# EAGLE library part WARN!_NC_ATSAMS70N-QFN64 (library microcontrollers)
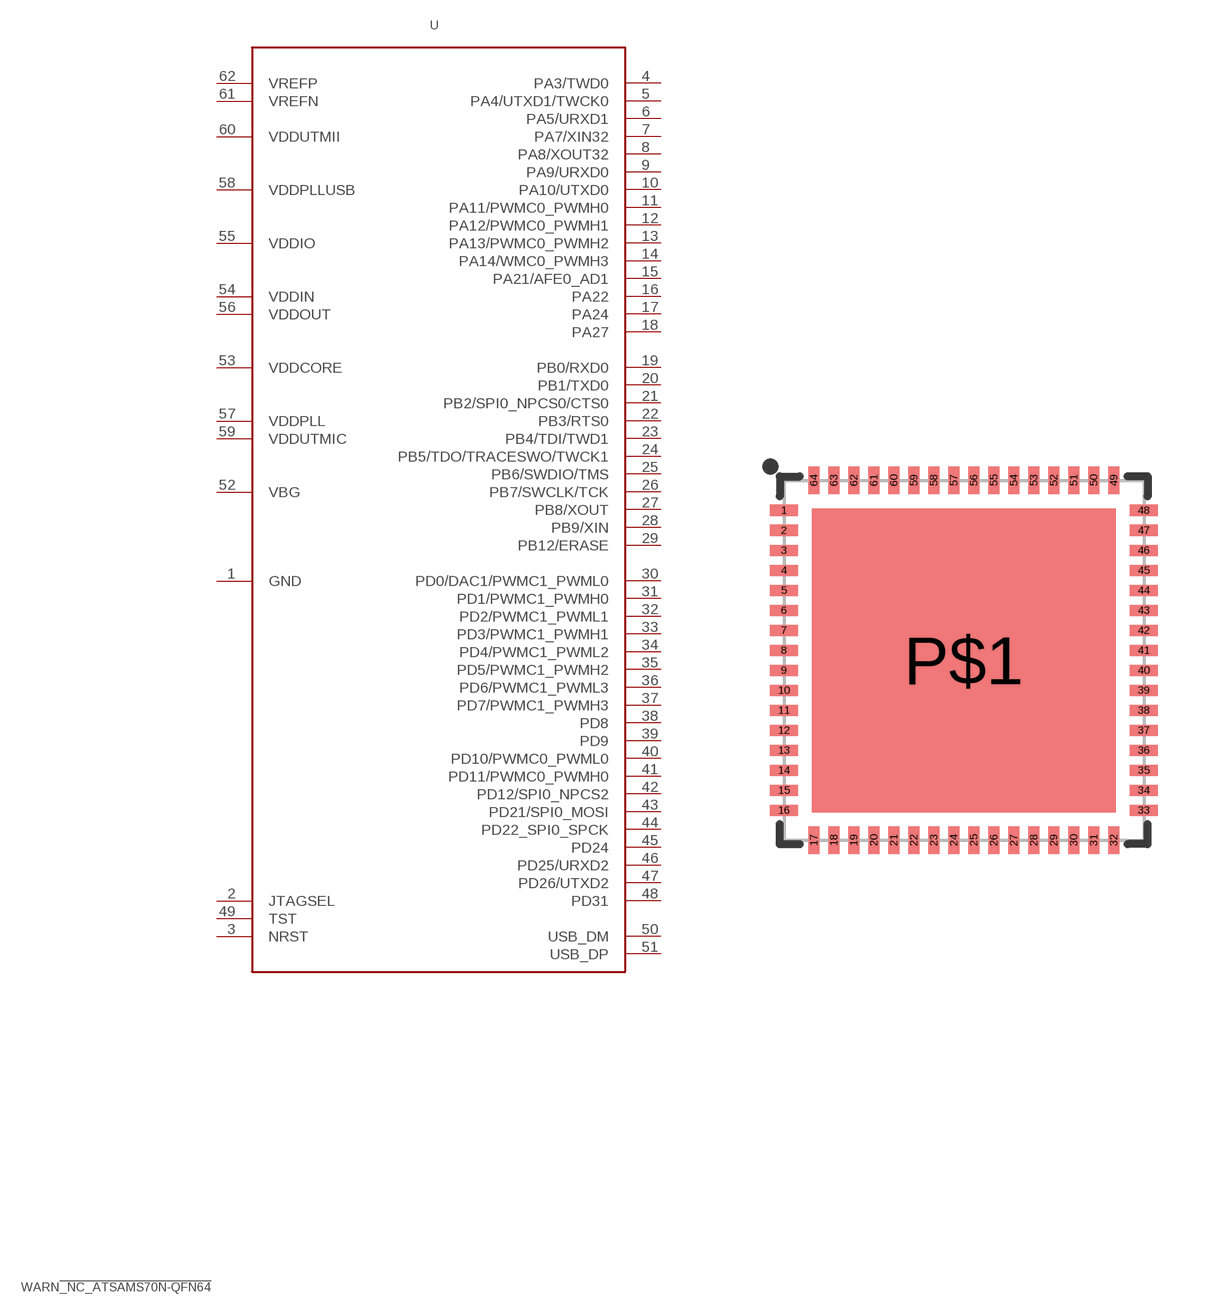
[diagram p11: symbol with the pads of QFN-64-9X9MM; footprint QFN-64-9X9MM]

Designator prefix U

## WARN!_NC_ATSAMS70N-QFN64  [QFN-64-9X9MM]
1  GND
2  JTAGSEL
3  NRST
4  PA3/TWD0
5  PA4/UTXD1/TWCK0
6  PA5/URXD1
7  PA7/XIN32
8  PA8/XOUT32
9  PA9/URXD0
10  PA10/UTXD0
11  PA11/PWMC0_PWMH0
12  PA12/PWMC0_PWMH1
13  PA13/PWMC0_PWMH2
14  PA14/WMC0_PWMH3
15  PA21/AFE0_AD1
16  PA22
17  PA24
18  PA27
19  PB0/RXD0
20  PB1/TXD0
21  PB2/SPI0_NPCS0/CTS0
22  PB3/RTS0
23  PB4/TDI/TWD1
24  PB5/TDO/TRACESWO/TWCK1
25  PB6/SWDIO/TMS
26  PB7/SWCLK/TCK
27  PB8/XOUT
28  PB9/XIN
29  PB12/ERASE
30  PD0/DAC1/PWMC1_PWML0
31  PD1/PWMC1_PWMH0
32  PD2/PWMC1_PWML1
33  PD3/PWMC1_PWMH1
34  PD4/PWMC1_PWML2
35  PD5/PWMC1_PWMH2
36  PD6/PWMC1_PWML3
37  PD7/PWMC1_PWMH3
38  PD8
39  PD9
40  PD10/PWMC0_PWML0
41  PD11/PWMC0_PWMH0
42  PD12/SPI0_NPCS2
43  PD21/SPI0_MOSI
44  PD22_SPI0_SPCK
45  PD24
46  PD25/URXD2
47  PD26/UTXD2
48  PD31
49  TST
50  USB_DM
51  USB_DP
52  VBG
53  VDDCORE
54  VDDIN
55  VDDIO
56  VDDOUT
57  VDDPLL
58  VDDPLLUSB
59  VDDUTMIC
60  VDDUTMII
61  VREFN
62  VREFP

## Footprint QFN-64-9X9MM (pad centres in mm)
64-pin QFN 9x9mm, 0.5mm pitch Package used by ATmega128RFA1 Example Datasheet
smd 0.7 x 0.275: 1 -4.5,3.75; 2 -4.5,3.25; 3 -4.5,2.75; 4 -4.5,2.25; 5 -4.5,1.75; 6 -4.5,1.25; 7 -4.5,0.75; 8 -4.5,0.25; 9 -4.5,-0.25; 10 -4.5,-0.75; 11 -4.5,-1.25; 12 -4.5,-1.75; 13 -4.5,-2.25; 14 -4.5,-2.75; 15 -4.5,-3.25; 16 -4.5,-3.75; 33 4.5,-3.75; 34 4.5,-3.25; 35 4.5,-2.75; 36 4.5,-2.25; 37 4.5,-1.75; 38 4.5,-1.25; 39 4.5,-0.75; 40 4.5,-0.25; 41 4.5,0.25; 42 4.5,0.75; 43 4.5,1.25; 44 4.5,1.75; 45 4.5,2.25; 46 4.5,2.75; 47 4.5,3.25; 48 4.5,3.75
smd 0.275 x 0.7: 17 -3.75,-4.5; 18 -3.25,-4.5; 19 -2.75,-4.5; 20 -2.25,-4.5; 21 -1.75,-4.5; 22 -1.25,-4.5; 23 -0.75,-4.5; 24 -0.25,-4.5; 25 0.25,-4.5; 26 0.75,-4.5; 27 1.25,-4.5; 28 1.75,-4.5; 29 2.25,-4.5; 30 2.75,-4.5; 31 3.25,-4.5; 32 3.75,-4.5; 49 3.75,4.5; 50 3.25,4.5; 51 2.75,4.5; 52 2.25,4.5; 53 1.75,4.5; 54 1.25,4.5; 55 0.75,4.5; 56 0.25,4.5; 57 -0.25,4.5; 58 -0.75,4.5; 59 -1.25,4.5; 60 -1.75,4.5; 61 -2.25,4.5; 62 -2.75,4.5; 63 -3.25,4.5; 64 -3.75,4.5
smd 7.6 x 7.6: P$1 0,0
